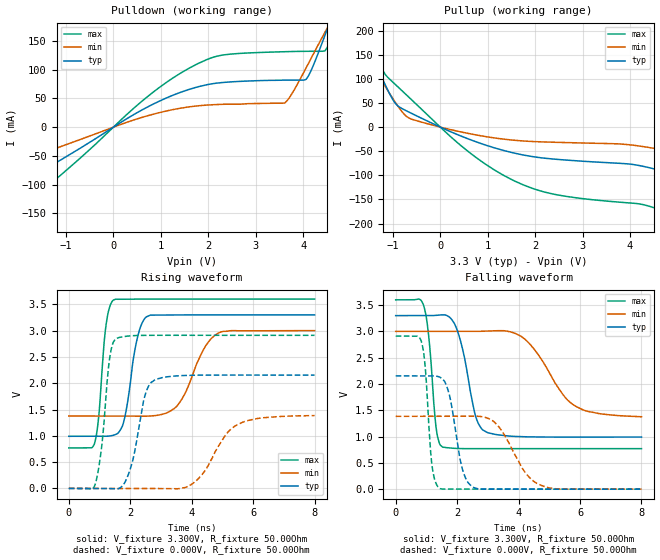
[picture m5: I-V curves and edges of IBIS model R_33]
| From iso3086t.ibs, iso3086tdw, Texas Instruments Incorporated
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|   R_33 MODEL
[Model]   R_33
Model_type   3-state
Polarity   Non-Inverting
Enable   Active-Low
Vmeas   = 1.65V
Vref   = 0V
Cref   = 15pF
|Average   typ   min   max
|   (Slow PVT)   (Nom PVT)   (fast PVT)
C_comp   2.0113872pF 2.0112967pF   2.0220429pF
| HIGH STATE   (Slow PVT)  (Nom PVT)   (Fast PVT )
|C_comp   2.0573842pF 2.0532906pF   2.0786956pF
| LOW STATE   (Nom PVT)   (Fast PVT)   (Slow PVT)
|C_comp   1.9633518pF 1.9693027pF   1.9653902pF
[Model Spec]
Vmeas   1.65V   1.5V   1.8V
[Voltage Range]   3.3   3.0   3.6
[Temperature Range]   40   125   -40
[Pullup Reference]   3.3   3.0   3.6
[Pulldown Reference]   0   0   0
[Power Clamp Reference]   3.3   3.0   3.6
[GND Clamp Reference]   0   0   0
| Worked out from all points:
|   slope of the pulldown table from 0 to 0.495 V, typ, clamps not added: 19.8 ohm
|   slope of the pullup table from 0 to 0.495 V, typ, clamps not added: 23.8 ohm
|   falling waveform, V_fixture 3.300V, R_fixture 50.00Ohm: 20-80 % time 469ps typ, 1.09ns min, 234ps max; typ from 3.3 V to 0.991 V
|   rising waveform, V_fixture 3.300V, R_fixture 50.00Ohm: 20-80 % time 365ps typ, 736ps min, 227ps max; typ from 0.991 V to 3.3 V
|   rising waveform, V_fixture 0.000V, R_fixture 50.00Ohm: 20-80 % time 427ps typ, 886ps min, 274ps max; typ from 0 V to 2.15 V
|   falling waveform, V_fixture 0.000V, R_fixture 50.00Ohm: 20-80 % time 374ps typ, 817ps min, 197ps max; typ from 2.15 V to 0 V
[Pulldown]
|   Voltage   I(typ)   I(min)   I(max)
-3.3V     -156.1mA   -96.61mA   -221.6mA
-2.355V   -115.1mA   -70.06mA   -165.3mA
-1.111V   -57.16mA   -33.9mA    -83.57mA
729.6mV   35.57mA    20.04mA    53.92mA
1.973V    73.97mA    38.46mA    117.9mA
2.471V    78.87mA    40.01mA    127.3mA
3.615V    81.88mA    42.2mA     131.5mA
4.063V    83.3mA     103.4mA    132.2mA
4.461V    160.3mA    165.6mA    133.1mA
4.56V     182.4mA    180.5mA    150.8mA
4.66V     204.5mA    195.1mA    179.9mA
6.6V      528.1mA    382.8mA    734.1mA
[Pullup]
|   Voltage   I(typ)   I(min)   I(max)
-3.3V     454.7mA    333.3mA    659mA
-2.007V   265.6mA    208.9mA    359mA
-1.708V   205.6mA    168mA      267.5mA
-1.509V   163.2mA    138.5mA    204.1mA
-1.211V   98.2mA     92mA       117.5mA
-862.3mV  41.64mA    39.05mA    80.56mA
-613.6mV  28.91mA    16.85mA    57.52mA
580.4mV   -24.07mA   -12.88mA   -49.92mA
1.725V    -57.3mA    -28.55mA   -118.7mA
4.262V    -80.97mA   -40.13mA   -160.4mA
5.555V    -117.5mA   -64.46mA   -209.4mA
6.6V      -153.8mA   -88.63mA   -257.4mA
[Ramp]
R_load = 50.00Ohm
|   typ   min   max
dV/dt_r   1.293V/426.515ps 830.974mV/885.638ps   1.746V/274.333ps
dV/dt_f   1.385V/469.113ps 973.889mV/1.094ns   1.698V/233.594ps
[Falling Waveform]
V_fixture = 3.300V
V_fixture_min = 3.000V
V_fixture_max = 3.600V
R_fixture = 50.00Ohm
|   Time   V(typ)   V(min)   V(max)
0s        3.3V       3V         3.6V
910ps     3.3V       3V         3.492V
1.08ns    3.3V       3V         2.88V
1.32ns    3.305V     3V         1.148V
1.52ns    3.315V     3V         803.1mV
2.01ns    3.01V      3V         773.5mV
2.85ns    1.12V      3.003V     769.7mV
4.18ns    996.1mV    2.865V     770.2mV
5.86ns    990.3mV    1.576V     770.3mV
8ns       991mV      1.377V     770.3mV
[Rising Waveform]
V_fixture = 3.300V
V_fixture_min = 3.000V
V_fixture_max = 3.600V
R_fixture = 50.00Ohm
|   Time   V(typ)   V(min)   V(max)
0s        991mV      1.377V     770.3mV
840ps     990.5mV    1.377V     860.8mV
1.2ns     991mV      1.377V     3.055V
1.45ns    1.01V      1.376V     3.581V
1.77ns    1.23V      1.376V     3.597V
2.21ns    2.807V     1.373V     3.6V
2.53ns    3.263V     1.373V     3.6V
3.51ns    3.299V     1.56V      3.6V
4.87ns    3.3V       2.954V     3.6V
8ns       3.3V       3V         3.6V
[Rising Waveform]
V_fixture = 0.000V
V_fixture_min = 0.000V
V_fixture_max = 0.000V
R_fixture = 50.00Ohm
|   Time   V(typ)   V(min)   V(max)
0s        28.97uV    34.06uV    23.08uV
860ps     302.9uV    115.5uV    80.51mV
1.33ns    -3.967mV   129.5uV    2.48V
1.54ns    -9.22mV    115.6uV    2.851V
1.96ns    299.7mV    216.8uV    2.899V
2.47ns    1.747V     -27.22uV   2.91V
2.8ns     2.063V     -1.454mV   2.911V
4.07ns    2.152V     109mV      2.911V
5.63ns    2.155V     1.251V     2.911V
8ns       2.154V     1.385V     2.911V
[Falling Waveform]
V_fixture = 0.000V
V_fixture_min = 0.000V
V_fixture_max = 0.000V
R_fixture = 50.00Ohm
|   Time   V(typ)   V(min)   V(max)
0s        2.154V     1.385V     2.911V
840ps     2.154V     1.385V     2.8V
970ps     2.155V     1.385V     2.256V
1.18ns    2.156V     1.385V     458.6mV
1.43ns    2.133V     1.385V     14.39mV
1.75ns    1.787V     1.385V     1.991mV
2.19ns    344.2mV    1.387V     38.79uV
2.52ns    36.58mV    1.39V      -99.04uV
4.67ns    -11.41uV   87.82mV    28.84uV
8ns       28.97uV    34.06uV    23.08uV
